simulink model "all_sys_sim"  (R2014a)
settings: Solver=ode45  StartTime=0.0  StopTime=10.0  RelTol=1e-3
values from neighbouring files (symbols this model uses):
  build_sys = sys_class    [create_all_sys.m]
  fom_sys = sys_class    [create_all_sys.m]
  heli_sys = sys_class    [create_all_sys.m]
  iss_sys = sys_class    [create_all_sys.m]
  mcs_sys = sys_class    [create_all_sys.m]
  pde_sys = sys_class    [create_all_sys.m]
  tline_sys = sys_class    [create_all_sys.m]

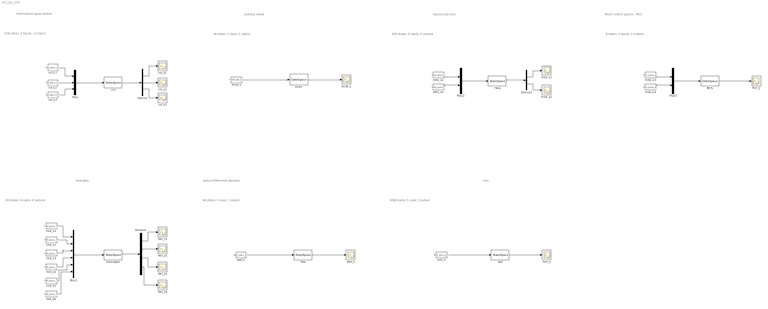
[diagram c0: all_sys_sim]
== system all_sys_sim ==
  note: 48 states, 1 input, 1 output
  note: 256 states, 3 inputs, 3 outputs
  note: 84 states, 1 input, 1 output
  note: 28 states, 6 inputs, 6 outputs
  note: 256 states, 2 inputs, 2 outputs
  note: 1006 states, 1 input, 1 output
  note: international space station
  note: building model
  note: helicopter
  note: partial differential equation
  note: fom
  note: transmission line
  note: 8 states, 2 inputs, 1 outputs
  note: Motor control system - MCS
  Build : StateSpace  A=build_sys.sys.a  B=build_sys.sys.b  C=build_sys.sys.c  D=build_sys.sys.d  X0=build_sys.x0_lb
  Demux : Demux  Outputs=3
  Demux1 : Demux
  Demux2 : Demux  Outputs=2
  Helicopter : StateSpace  A=heli_sys.sys.a  B=heli_sys.sys.b  C=heli_sys.sys.c  D=heli_sys.sys.d  X0=heli_sys.x0_lb
  ISS : StateSpace  A=iss_sys.sys.a  B=iss_sys.sys.b  C=iss_sys.sys.c  D=iss_sys.sys.d  X0=iss_sys.x0_lb
  MCS : StateSpace  A=mcs_sys.sys.a  B=mcs_sys.sys.b  C=mcs_sys.sys.c  D=mcs_sys.sys.d  X0=mcs_sys.x0_lb
  Mux : Mux  Inputs=3
  Mux1 : Mux  Inputs=6
  Mux2 : Mux  Inputs=2
  Mux3 : Mux  Inputs=2
  Pde : StateSpace  A=pde_sys.sys.a  B=pde_sys.sys.b  C=pde_sys.sys.c  D=pde_sys.sys.d  X0=pde_sys.x0_lb
  Tline : StateSpace  A=tline_sys.sys.a  B=tline_sys.sys.b  C=tline_sys.sys.c  D=tline_sys.sys.d  X0=tline_sys.x0_lb
  build_u : Constant  Value=build_sys.u_ub(1)
  build_y : Scope
  fom : StateSpace  A=fom_sys.sys.a  B=fom_sys.sys.b  C=fom_sys.sys.c  D=fom_sys.sys.d  X0=fom_sys.x0_lb
  fom_u : Constant  Value=fom_sys.u_ub(1)
  fom_y : Scope
  heli_u1 : Constant  Value=heli_sys.u_ub(1)
  heli_u2 : Constant  Value=heli_sys.u_ub(2)
  heli_u3 : Constant  Value=heli_sys.u_ub(3)
  heli_u4 : Constant  Value=heli_sys.u_ub(4)
  heli_u5 : Constant  Value=heli_sys.u_ub(5)
  heli_u6 : Constant  Value=heli_sys.u_ub(6)
  heli_y{1..4} (4 alike) : Scope
  iss_u1 : Constant  Value=iss_sys.u_ub(1)
  iss_u2 : Constant  Value=iss_sys.u_ub(2)
  iss_u3 : Constant  Value=iss_sys.u_ub(3)
  iss_y1 : Scope
  iss_y2 : Scope
  iss_y3 : Scope
  mcs_y : Scope
  pde_u : Constant  Value=pde_sys.u_ub(1)
  pde_y : Scope
  tline_u1 : Constant  Value=tline_sys.u_ub(1)
  tline_u2 : Constant  Value=tline_sys.u_ub(2)
  tline_u3 : Constant  Value=mcs_sys.u_ub(1)
  tline_u4 : Constant  Value=mcs_sys.u_ub(2)
  tline_y1 : Scope
  tline_y2 : Scope
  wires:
  Mux/1 -> ISS/1
  iss_u1/1 -> Mux/1
  iss_u2/1 -> Mux/2
  iss_u3/1 -> Mux/3
  ISS/1 -> Demux/1
  Demux/1 -> iss_y1/1
  Demux/2 -> iss_y2/1
  Demux/3 -> iss_y3/1
  build_u/1 -> Build/1
  Build/1 -> build_y/1
  heli_u1/1 -> Mux1/1
  heli_u2/1 -> Mux1/2
  heli_u3/1 -> Mux1/3
  Mux1/1 -> Helicopter/1
  heli_u4/1 -> Mux1/4
  heli_u5/1 -> Mux1/5
  heli_u6/1 -> Mux1/6
  Helicopter/1 -> Demux1/1
  pde_u/1 -> Pde/1
  Pde/1 -> pde_y/1
  Mux2/1 -> Tline/1
  tline_u1/1 -> Mux2/1
  tline_u2/1 -> Mux2/2
  Tline/1 -> Demux2/1
  Demux2/1 -> tline_y1/1
  Demux2/2 -> tline_y2/1
  fom_u/1 -> fom/1
  fom/1 -> fom_y/1
  Demux1/1 -> heli_y1/1
  Demux1/2 -> heli_y2/1
  Demux1/3 -> heli_y3/1
  Demux1/4 -> heli_y4/1
  Mux3/1 -> MCS/1
  tline_u3/1 -> Mux3/1
  tline_u4/1 -> Mux3/2
  MCS/1 -> mcs_y/1
